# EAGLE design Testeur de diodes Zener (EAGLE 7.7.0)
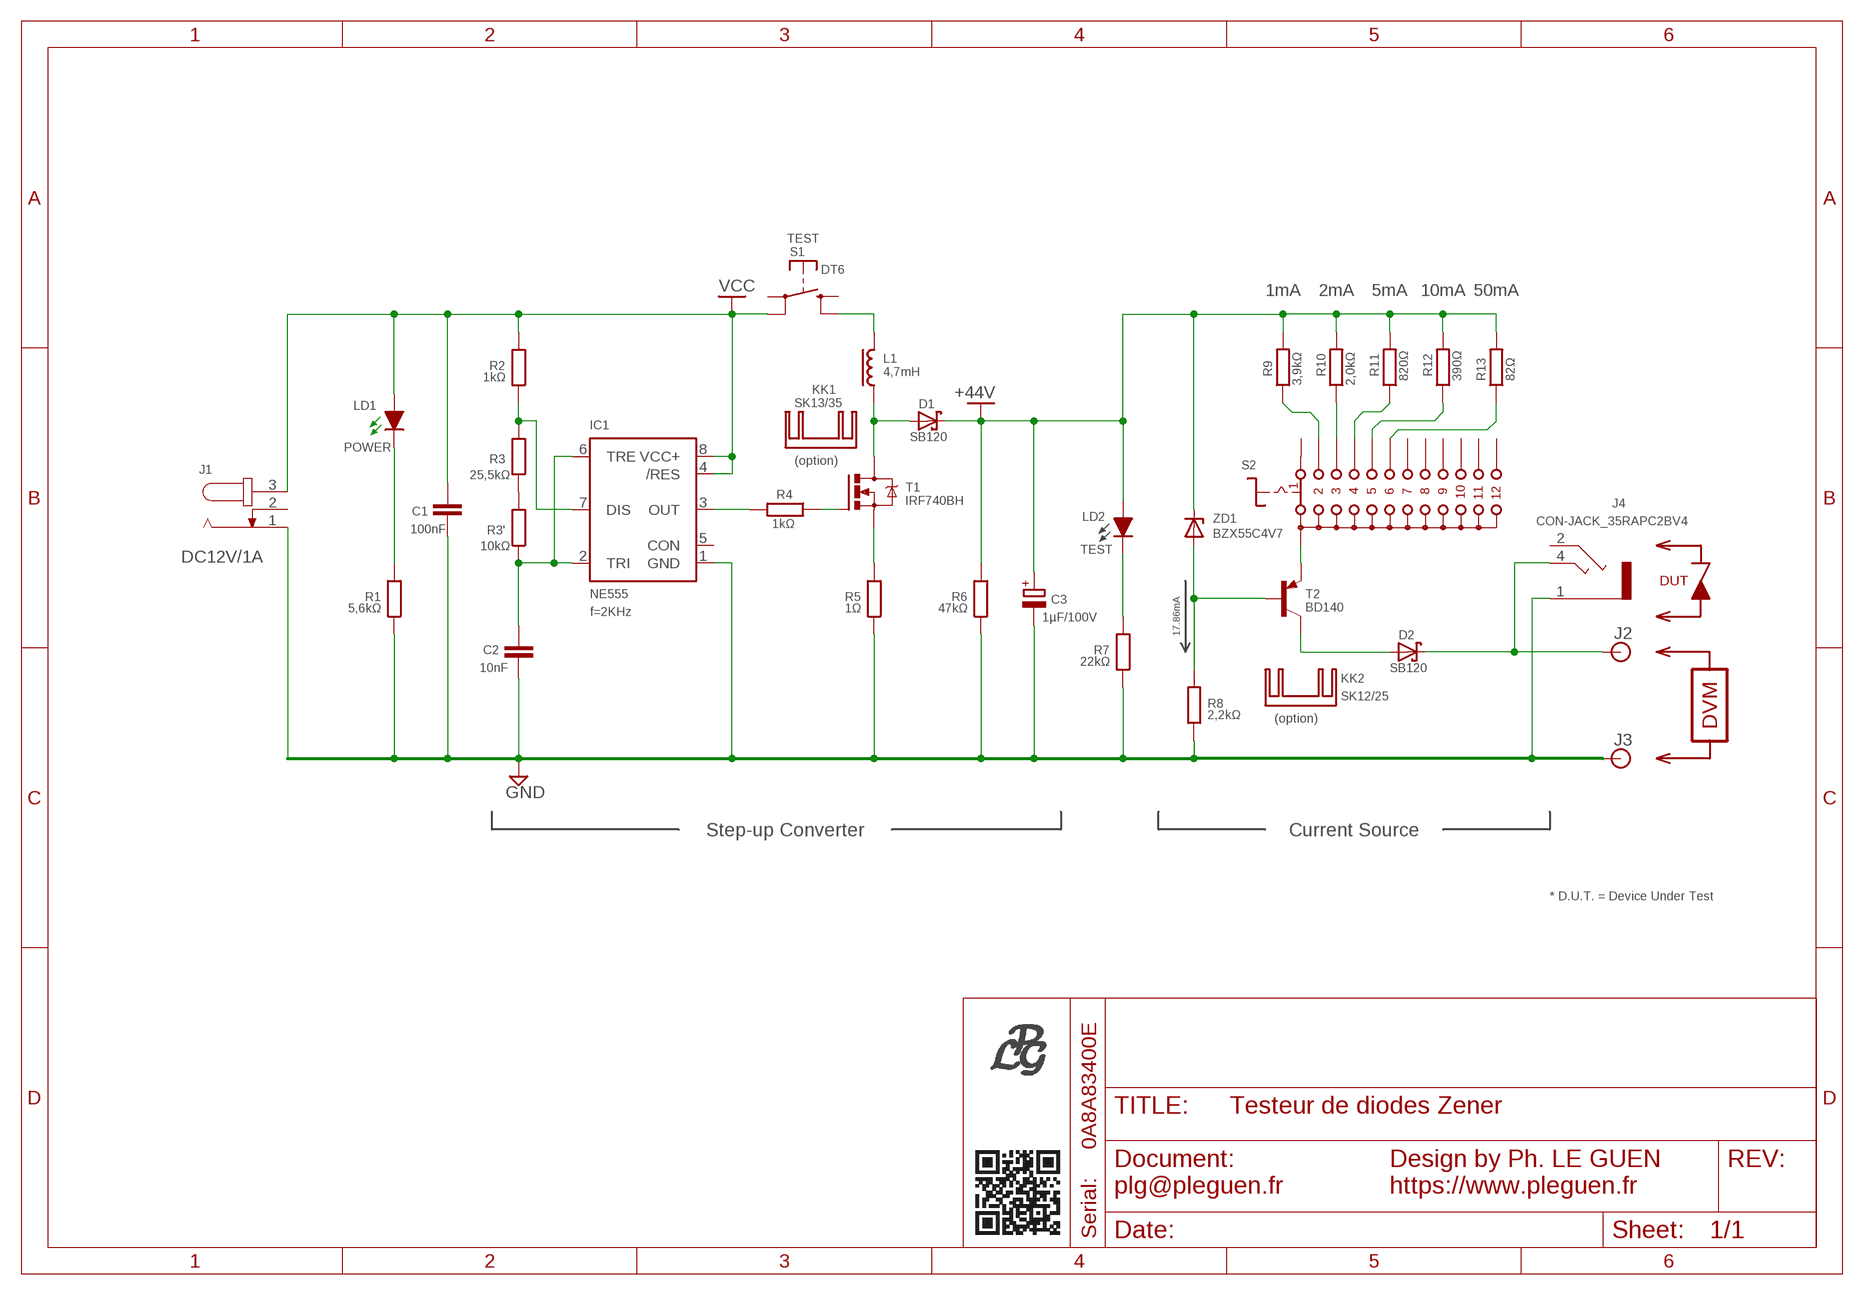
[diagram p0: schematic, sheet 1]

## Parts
C1  100nF  C-EU025-024X044  [C025-024X044]
C2  10nF  C-EU025_050-025X075  [C025_050-025X075]
C3  1µF/100V  CPOL-EUE2.5-5  [E2,5-5]
D1  SB120  [DO41-10]
D2  SB120  [DO41-10]
IC1  NE555  [DIL-08]
J1  DC12V/1A  JACK-PLUG0  [SPC4077]
J2  BANANA_CONN  [BANANA_CONN]
J3  BANANA_CONN  [BANANA_CONN]
J4  CON-JACK_35RAPC2BV4  [CON-JACK_35RAPC2BV4]
KK1  SK13/35  [SK13/35]
KK2  SK12/25  [SK12/25]
L1  4,7mH  L-RL8XX  [RL8XX]
LD1  LED_3MM_GREEN  [LED_3MM]
LD2  LED_3MM_WHITE  [LED_3MM]
R1  5,6kΩ  R-EU_0207/7  [0207/7]
R2  1kΩ  R-EU_0207/7  [0207/7]
R3  25,5kΩ  R-EU_0207/7  [0207/7]
R3'  10kΩ  R-EU_0207/7  [0207/7]
R4  1kΩ  R-EU_0207/7  [0207/7]
R5  1Ω  R-EU_0207/7  [0207/7]
R6  47kΩ  R-EU_0207/7  [0207/7]
R7  22kΩ  R-EU_0207/7  [0207/7]
R8  2,2kΩ  R-EU_0207/7  [0207/7]
R9  3,9kΩ  R-EU_0207/7  [0207/7]
R10  2,0kΩ  R-EU_0207/7  [0207/7]
R11  820Ω  R-EU_0207/7  [0207/7]
R12  390Ω  R-EU_0207/7  [0207/7]
R13  82Ω  R-EU_0207/7  [0207/7]
S1  DT6  [DT6]
S2  CK101X12  [CK101X12]
T1  IRF740BH  [TO220BH]
T2  BD140  [TO126]
ZD1  BZX55C4V7  ZENER-DIODEZD-7.5  [ZDIO-7.5]

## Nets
+48V [POWER]: C3.+ D1.C LD2.A R6.2 R9.2 R10.2 R11.2 R12.2 R13.2 ZD1.C ; supply symbol labelled +44V
GND: C1.2 C2.1 C3.- IC1.1(GND) J1.1 J3.P$1 J4.1 R1.1 R5.1 R6.1 R7.1 R8.1
N$1: C2.2 IC1.2(TRI) IC1.6(TRE) R3'.1
N$2 [POWER]: R12.1 S2.5
N$3 [POWER]: R11.1 S2.4
N$4 [POWER]: R9.1 S2.2
N$5: LD1.K(C) R1.2
N$6 [POWER]: R13.1 S2.6
N$7: IC1.7(DIS) R2.1 R3.2
N$8 [POWER]: S2.A T2.1(E)
N$9: R8.2 T2.3(B) ZD1.A
N$10: LD2.K(C) R7.2
N$11 [VCC]: L1.2 S1.2(S)
N$12: IC1.3(OUT) R4.2
N$13: R3'.2 R3.1
N$14 [POWER]: R5.2 T1.S
N$15: R4.1 T1.G
N$16 [VCC]: D1.A L1.1 T1.D
N$17 [POWER]: D2.A T2.2(C)
N$19 [POWER]: D2.C J2.P$1 J4.4
N$21 [POWER]: R10.1 S2.3
VCC [VCC]: C1.1 IC1.4(/RES) IC1.8(VCC+) J1.3 LD1.A R2.2 S1.4(P)
Unconnected: IC1.5(CON) J1.2 J4.2 S1.1(S) S1.3(P) S2.1 S2.7 S2.8 S2.9 S2.10 S2.11 S2.12

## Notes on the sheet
- TEST
- 1mA | 2mA | 5mA | 10mA | 50mA
- POWER
- (option)
- TEST
- DUT
- f=2KHz | 17.86mA
- DVM
- (option)
- Step-up Converter | Current Source
- * D.U.T. = Device Under Test
- 0A8A83400E

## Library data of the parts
C1 C2 = rcl:C-EU: CAPACITOR, European symbol
C3 = rcl:CPOL-EU: POLARIZED CAPACITOR, European symbol
D1 D2 = diode:SB120: DIODE
IC1 = st-microelectronics:NE555: General purpose bipolar Timer; MF: Arrow Electronics; MPN: NE555N; OC_FARNELL: 1467742; OC_NEWARK: 89K1486
J1 = Library_PLG:JACK-PLUG: DC POWER JACK Power Jack, DC, Right Angle, Through Hole, Rated 5A at 16VDC, PC Terminals Distributor: Farnell (www.Farnell.de) Drawing: 84N1161.pdf / 84N1162.pdf Manufacturer: SPC Technology (www.spctechnology.com) Type: SPC4077 / SPC 4078; OC_FARNELL: 1654842; OC_NEWARK: unknown
J2 J3 = SparkFun-Connectors:BANANA_CONN: Through-hole Banana Jack
J4 = Library_PLG:CON-JACK_35RAPC2BV4: Klinkensteckverbinder nach JISC 6560, 2,5 mm Jack connectors according to JISC 6560, 2.5 mm Source: http://www.lumberg.com/Produkte/PDFs/1501_03.pdf
KK1 = heatsink:SK13/35: HEATSINK
KK2 = heatsink:SK12/25: HEATSINK
L1 = inductors-jwmiller:L: INDUCTORS
LD1 = Library_PLG:LED_3MM_GREEN
LD2 = Library_PLG:LED_3MM_WHITE
R1-R3 R3' R4-R13 = rcl:R-EU_: RESISTOR, European symbol
S1 = switch-misc:DT: ITT SWITCH
S2 = Library_PLG:CK101X12: ROTARY SWITCH C&K
T1 = transistor-power:IRF740: N-CHANNEL MOS FET
T2 = transistor-pnp:BD140: PNP Transistor
ZD1 = diode:ZENER-DIODE: Z-Diode

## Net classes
1 POWER: width 0.813 mm, clearance 0.61 mm
2 VCC: width 0.813 mm, clearance 0.508 mm

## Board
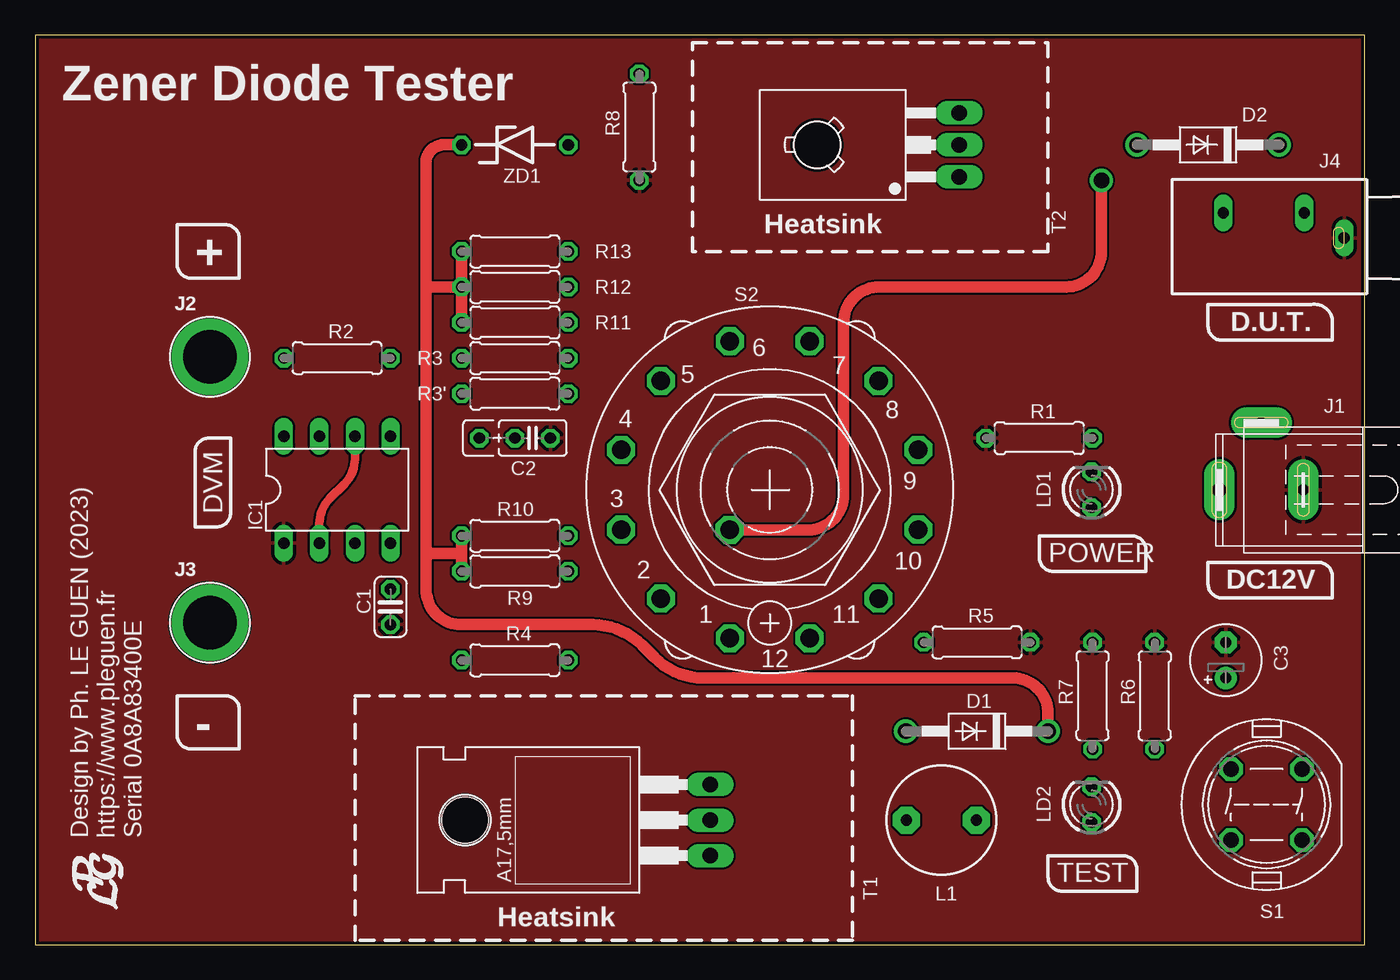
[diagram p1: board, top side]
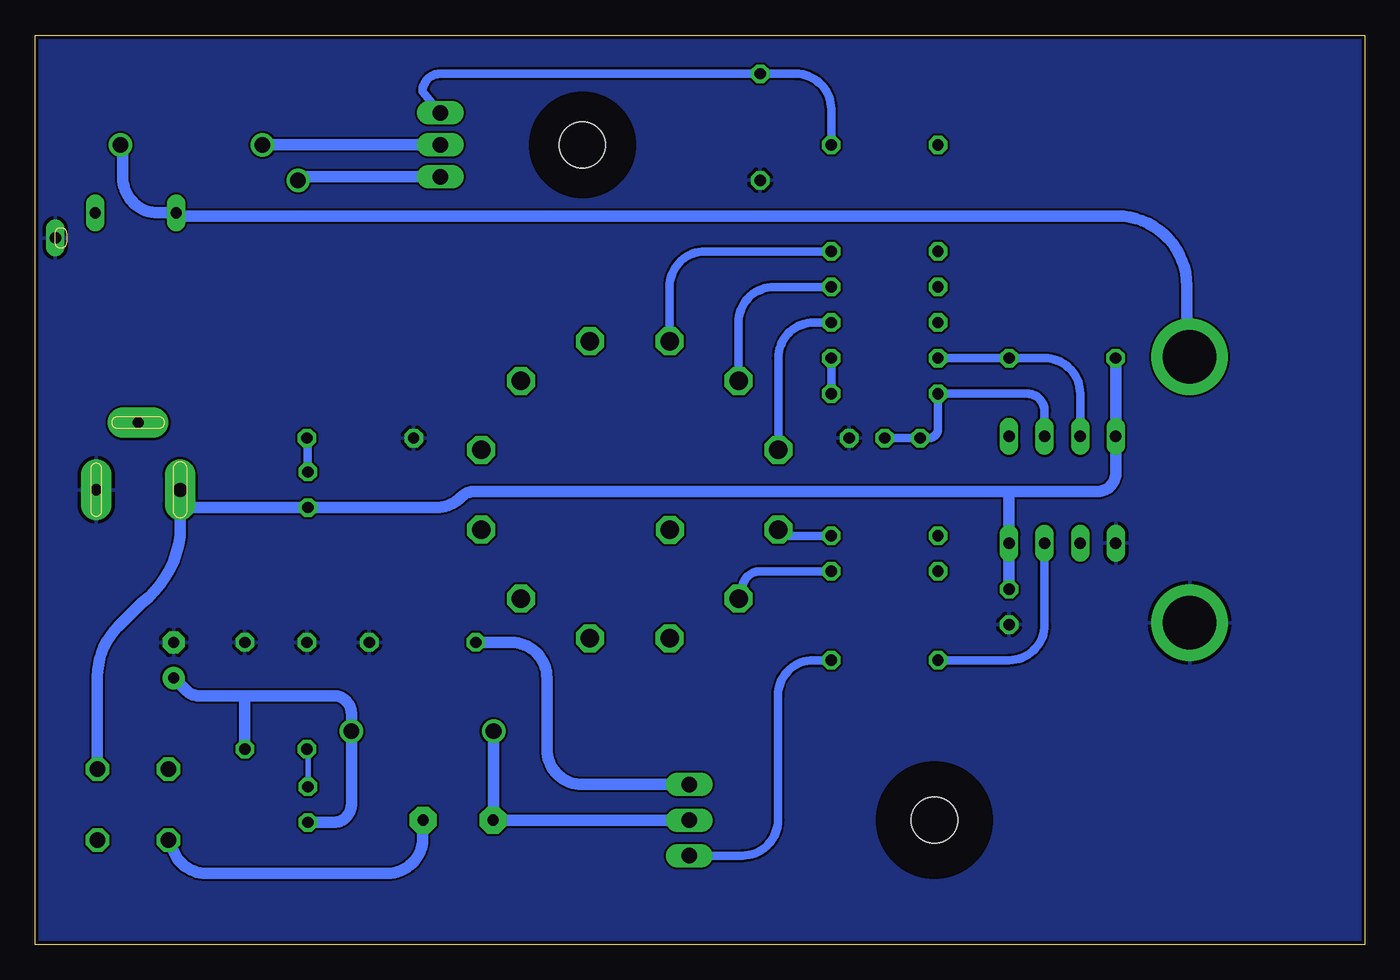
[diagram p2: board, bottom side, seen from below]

Size 95 x 65 mm. Coordinates in mm from the lower left corner, seen from the top.
Outline: 0,0 95,0 95,65 0,65 0,0
Copper layers (1*16): Top 0.035mm / dielectric 1.5mm / Bottom 0.035mm
Design rules "SeeedStudio_2layer_DRU_no_angle_20140221": minimum track width 6mil, minimum drill 12mil, track to track 6mil, track to pad 6mil, pad to pad 6mil, via to via 6mil, smd to smd 0mil, copper to edge 10mil, drill to drill 10mil, minimum pad ring 10mil, minimum via ring 6mil, stop-mask expansion 2mil, vias tented up to drill 100mil, thermal gap 10mil

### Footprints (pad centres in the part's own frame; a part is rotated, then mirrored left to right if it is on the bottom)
C025-024X044 = drill 0.813 octagon: 1 -1.27,0; 2 1.27,0
C025_050-025X075 = drill 0.813 octagon: 1 -1.27,0; 2 1.27,0; 3 3.81,0
E2,5-5 = drill 0.813 pad 1.6: + -1.27,0 | drill 0.813 pad 1.6 octagon: - 1.27,0
DO41-10 = drill 1.118: A 5.08,0; C -5.08,0
DIL-08 = drill 0.813 long: 1 -3.81,-3.81; 2 -1.27,-3.81; 3 1.27,-3.81; 4 3.81,-3.81; 5 3.81,3.81; 6 1.27,3.81; 7 -1.27,3.81; 8 -3.81,3.81
SPC4077 = drill 0.8 pad 2.184 long: 1 -3,0; 2 0,-4.8 | drill 1 pad 2.184 long: 3 3,0
BANANA_CONN = drill 3.81 pad 5.461: P$1 0,0
CON-JACK_35RAPC2BV4 = drill 0.8 pad 1.2 long: 1 0,-1.71; 2 -1.79,-4.55; 4 -1.79,-10.33
RL8XX = drill 0.813 pad 1.93 octagon: 1 -2.5,0; 2 2.5,0
LED_3MM = drill 0.813 octagon: A -1.27,0; K 1.27,0
0207/7 = drill 0.813 octagon: 1 -3.81,0; 2 3.81,0
DT6 = drill 1.118 octagon: 1 -2.54,2.54; 2 2.54,2.54; 3 2.54,-2.54; 4 -2.54,-2.54
CK101X12 = drill 1.321 octagon: 1 -2.845,-10.617; 2 -7.772,-7.772; 3 -10.617,-2.845; 4 -10.617,2.845; 5 -7.772,7.772; 6 -2.845,10.617; 7 2.845,10.617; 8 7.772,7.772; 9 10.617,2.845; 10 10.617,-2.845; 11 7.772,-7.772; 12 2.845,-10.617; A -2.87,-2.87
TO220BH = drill 1.118 long: D 0,-6.35; G -2.54,-6.35; S 2.54,-6.35 | hole 3.302: 0,11.176
TO126 = drill 1.118 long: 1 -2.286,-5.08; 2 0,-5.08; 3 2.286,-5.08 | hole 3.302: 0,5.08
ZDIO-7.5 = drill 0.813 octagon: A 3.81,0; C -3.81,0

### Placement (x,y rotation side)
C1  25.4,24.13 270 top
C2  35.56,36.2 180 top
C3  85.09,20.32 90 top
D1  67.31,15.24 180 top
D2  83.82,57.15 180 top
IC1  21.59,32.5 0 top
J1  87.63,32.5 180 top
J2  12.5,42 0 top
J3  12.5,23 0 top
J4  95.25,50.5 270 top
KK1  not placed on the board
KK2  not placed on the board
L1  64.77,8.89 0 top
LD1  75.5,32.5 90 top
LD2  75.5,10 90 top
R1  71.75,36.2 0 top
R2  21.59,41.91 180 top
R3  34.29,41.91 180 top
R3'  34.29,39.37 0 top
R4  34.29,20.32 180 top
R5  67.31,21.59 180 top
R6  80.01,17.78 270 top
R7  75.56,17.78 270 top
R8  43.18,58.42 90 top
R9  34.29,26.67 180 top
R10  34.29,29.21 180 top
R11  34.29,44.45 180 top
R12  34.29,46.99 180 top
R13  34.29,49.53 180 top
S1  88,10 180 top
S2  52.5,32.5 0 top
T1  41.91,8.89 90 top
T2  60.96,57.15 90 top
U$1  [LOGO_PLG]  6.35,2.54 90 top
ZD1  34.29,57.15 0 top

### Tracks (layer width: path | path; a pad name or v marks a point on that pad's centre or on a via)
+48V
  Top 0.813: R9.2 30.48,27.94 | 30.48,27.94 R10.2 | 27.94,46.99 27.94,27.94 | D1.C 72.39,16.51 arc90 69.85,19.05 47.79,19.05 arc-45 44.26,20.51 43.37,21.4 arc45 39.84,22.86 30.48,22.86 arc-90 27.94,25.4 27.94,27.94 | ZD1.C 29.21,57.15 arc90 27.94,55.88 27.94,46.99 | R13.2 R12.2 | R12.2 R11.2 | R12.2 27.94,46.99 | 30.48,27.94 27.94,27.94
  Bottom 0.813: LD2.A 73.66,8.73 arc-90 72.39,10 D1.C 72.39,16.51 arc-90 73.66,17.78 80.01,17.78 | C3.+ 84.19,18.15 arc-45 83.29,17.78 80.01,17.78 | 80.01,17.78 R6.2
GND
  pour Bottom: 0,0 95,0 95,65 0,65
  pour Top: 0,0 95,0 95,65 0,65
N$1
  Top 0.61: IC1.6 22.86,34.71 arc-45 22.12,32.91 21.06,31.86 arc45 20.32,30.06 IC1.2
  Bottom 0.61: IC1.6 22.86,38.1 arc-90 24.13,39.37 R3'.1 30.48,36.83 arc90 31.11,36.2 C2.2
N$2
  Bottom 0.61: R12.1 42.19,46.99 arc-90 44.73,44.45 S2.5
N$3
  Bottom 0.61: R11.1 39.34,44.45 arc-90 41.88,41.91 S2.4
N$4
  Bottom 0.61: R9.1 43.19,26.67 arc-73 44.41,25.77 S2.2
N$5
  Bottom 0.61: LD1.K 75.5,33.66 R1.2
N$6
  Bottom 0.61: R13.1 47.12,49.53 arc-90 49.66,46.99 S2.6
N$7
  Bottom 0.61: R3.2 R2.1 22.86,41.91 arc90 20.32,39.37 IC1.7
N$8  (via drill 1.1)
  Top 0.813: v76.2,54.61 76.2,49.53 arc-90 73.66,46.99 60.33,46.99 arc90 57.78,44.45 57.78,32.17 arc-90 55.24,29.63 S2.A
  Bottom 0.813: T2.1 76.2,54.86 v76.2,54.61
N$9
  Bottom 0.61: ZD1.A 38.1,59.69 arc-90 40.64,62.23 R8.2 66.04,62.23 arc-90 67.31,60.96 T2.3
N$10
  Bottom 0.406: R7.2 75.5,13.97 LD2.K
N$11
  Bottom 0.813: S1.2 85.3,7.62 85.28,7.41 arc-85 82.75,5.08 69.83,5.08 arc-89 67.29,7.58 L1.2
N$12
  Bottom 0.61: R4.2 25.4,20.32 arc-90 22.86,22.86 IC1.3
N$13
  Bottom 0.61: R3.1 R3'.2
N$14
  Bottom 0.813: T1.S 55.88,11.43 arc90 58.42,13.97 58.42,19.05 arc-90 60.96,21.59 R5.2
N$15
  Bottom 0.61: T1.G 44.45,6.35 arc-90 41.91,8.89 41.91,17.78 arc90 39.37,20.32 R4.1
N$16
  Bottom 0.813: T1.D L1.1 62.23,8.93 D1.A
N$17
  Bottom 0.813: D2.A T2.2
N$19
  Bottom 0.813: D2.C 88.73,57.15 88.73,54.83 arc-90 86.19,52.29 J4.4 | 85.09,52.29 J4.4 | J4.4 84.92,52.07 17.7,52.07 arc90 12.7,47.07 12.7,42 J2.P$1
N$21
  Bottom 0.61: R10.1 41.88,29.21 S2.3
VCC
  Bottom 0.813: J1.3 84.63,31.23 | 84.63,31.23 84.63,29.2 arc45 87.36,24.4 89.08,22.68 arc-45 90.54,19.15 S1.4 | 84.63,31.23 LD1.A 66.34,31.23 arc-45 64.55,31.97 arc45 63.55,32.38 25.4,32.38 | 25.4,32.38 19.05,32.38 arc-90 17.78,33.66 IC1.8 R2.2 | 25.4,32.38 IC1.4 C1.1

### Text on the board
tPlace: Zener Diode Tester | Heatsink | + | D.U.T. | DVM | POWER | DC12V | - | Design by Ph. LE GUEN (2023) / https://www.pleguen.fr / Serial 0A8A83400E | TEST | Heatsink

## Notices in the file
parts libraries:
supply0: Copyright (C) 2007, Bob Starr
SparkFun-Connectors: Licensing: Creative Commons ShareAlike 4.0 International - https://creativecommons.org/licenses/by-sa/4.0
